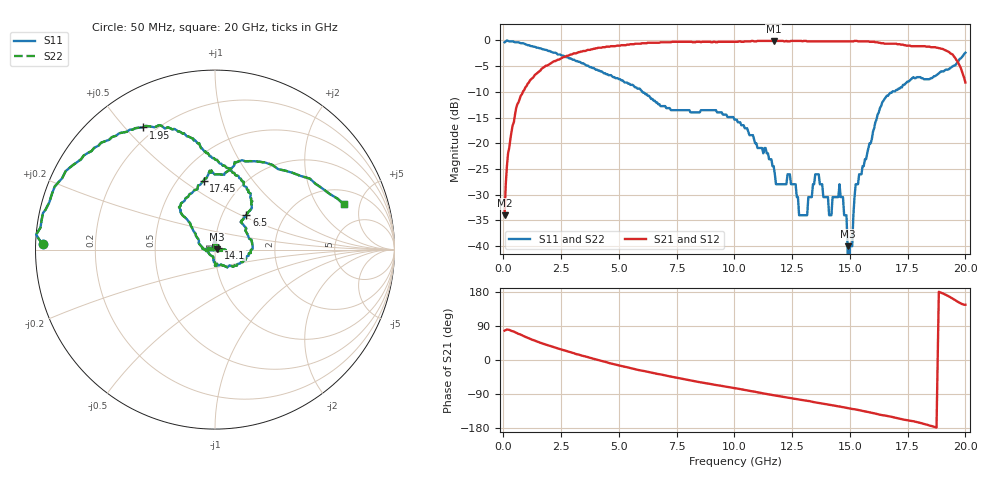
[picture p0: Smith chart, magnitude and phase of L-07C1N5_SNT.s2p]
#	mhz	s	ma	r	50
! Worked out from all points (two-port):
!   400 points, 50 MHz to 20 GHz, reference 50 ohm
!   highest |S21| = -0.09 dB at 11.7 GHz (marker M1); lowest = -34.0 dB at 50 MHz (marker M2)
!   |S21| within 3 dB of the highest: 2.704 GHz to 19.5 GHz (16.79 GHz wide, 151 % of centre)
!   lowest |S11| = -40.0 dB at 14.9 GHz (marker M3), VSWR 1.02, Z = 51 + j0.191 ohm
!   |S11| at or under -10 dB: 6.019 GHz to 16.83 GHz (10.81 GHz wide, 94.6 % of centre)
!   |S22| runs from - to 0.0 dB; largest |S21 - S12| = 0
!   S11 on the Smith chart (normalised r, x): 50 MHz: 0.02, +0.01; 1.95 GHz: 0.15, +0.56; 6.5 GHz: 1.30, +0.54; 14.1 GHz: 1.03, +0.02; 17.45 GHz: 0.66, +0.60; 20 GHz: 2.94, +3.51
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50  0.96 178.3  0.02 77.6  0.02 77.6  0.96 178.3
550  0.96 161.4  0.22 72.1  0.22 72.1  0.96 161.4
1950  0.79 120.5  0.58 38.4  0.58 38.4  0.79 120.5
3400  0.6 99.2  0.78 11.5  0.78 11.5  0.6 99.2
6500  0.26 47.7  0.95 -34.4  0.95 -34.4  0.26 47.7
6700  0.24 47.7  0.95 -37.0  0.95 -37.0  0.24 47.7
10050  0.17 -22.1  0.97 -74.6  0.97 -74.6  0.17 -22.1
11700  0.06 -98.3  0.99 -93.0  0.99 -93.0  0.06 -98.3
13350  0.03 104.4  0.98 -110.1  0.98 -110.1  0.03 104.4
13650  0.05 86.9  0.98 -113.4  0.98 -113.4  0.05 86.9
14100  0.02 32.2  0.98 -117.9  0.98 -117.9  0.02 32.2
14550  0.04 -10.3  0.98 -122.7  0.98 -122.7  0.04 -10.3
14900  0.01 10.8  0.98 -126.9  0.98 -126.9  0.01 10.8
14950  0 16.5  0.98 -127.5  0.98 -127.5  0 16.5
15000  0.01 91.1  0.98 -128.1  0.98 -128.1  0.01 91.1
15250  0.04 -176.0  0.99 -130.5  0.99 -130.5  0.04 -176.0
16700  0.3 130.6  0.93 -148.7  0.93 -148.7  0.3 130.6
17450  0.39 99.3  0.89 -158.5  0.89 -158.5  0.39 99.3
18750  0.46 78.7  0.85 -178.4  0.85 -178.4  0.46 78.7
18800  0.47 77.9  0.85 0.7  0.85 0.7  0.47 77.9
18850  0.48 77.2  0.84 179.9  0.84 179.9  0.48 77.2
20000  0.76 19.4  0.39 145.8  0.39 145.8  0.76 19.4
